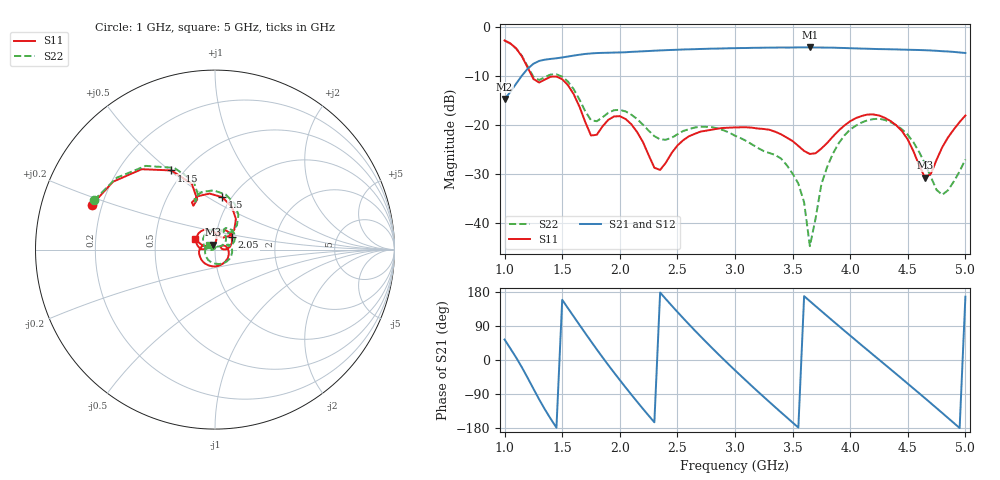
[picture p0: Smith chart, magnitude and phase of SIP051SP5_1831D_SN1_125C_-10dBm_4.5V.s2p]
# GHz  S  dB  R  50
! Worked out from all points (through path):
!   81 points, 1 GHz to 5 GHz, reference 50 ohm
!   highest |S21| = -4.13 dB at 3.65 GHz (marker M1); lowest = -14.7 dB at 1 GHz (marker M2)
!   lowest |S11| = -30.7 dB at 4.65 GHz (marker M3), VSWR 1.06, Z = 49 + j2.73 ohm
!   |S11| at or under -10 dB: 1.238 GHz to end of sweep
!   |S22| runs from -44.6 to -2.8 dB; largest |S21 - S12| = 0.0021
!   S11 on the Smith chart (normalised r, x): 1 GHz: 0.16, +0.17; 1.15 GHz: 0.43, +0.51; 1.5 GHz: 0.91, +0.58; 2.05 GHz: 1.19, +0.17; 5 GHz: 0.80, +0.10
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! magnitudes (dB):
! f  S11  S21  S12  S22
! 1 GHz  -2.7  -14.7  -14.6  -2.8
! 1.15 GHz  -6.0  -9.9  -9.9  -5.9
! 1.3 GHz  -11.3  -6.9  -6.9  -10.8
! 1.5 GHz  -10.6  -6.2  -6.2  -10.1
! 1.7 GHz  -19.3  -5.5  -5.5  -17.1
! 1.75 GHz  -22.1  -5.4  -5.3  -19.0
! 2.05 GHz  -18.7  -5.1  -5.1  -17.2
! 2.35 GHz  -29.1  -4.8  -4.7  -22.9
! 2.6 GHz  -22.2  -4.5  -4.5  -20.8
! 3 GHz  -20.4  -4.3  -4.3  -22.1
! 3.5 GHz  -23.2  -4.2  -4.2  -29.9
! 3.6 GHz  -25.2  -4.1  -4.1  -35.7
! 3.65 GHz  -25.8  -4.1  -4.1  -44.6
! 3.7 GHz  -25.7  -4.2  -4.1  -38.9
! 3.8 GHz  -23.6  -4.2  -4.2  -28.5
! 3.95 GHz  -20.0  -4.3  -4.3  -22.1
! 4.15 GHz  -17.8  -4.4  -4.4  -19.0
! 4.35 GHz  -19.1  -4.5  -4.5  -19.4
! 4.5 GHz  -22.9  -4.6  -4.6  -22.0
! 4.65 GHz  -30.7  -4.7  -4.7  -27.9
! 4.8 GHz  -24.4  -4.9  -4.9  -34.2
! 5 GHz  -18.0  -5.3  -5.3  -27.0
